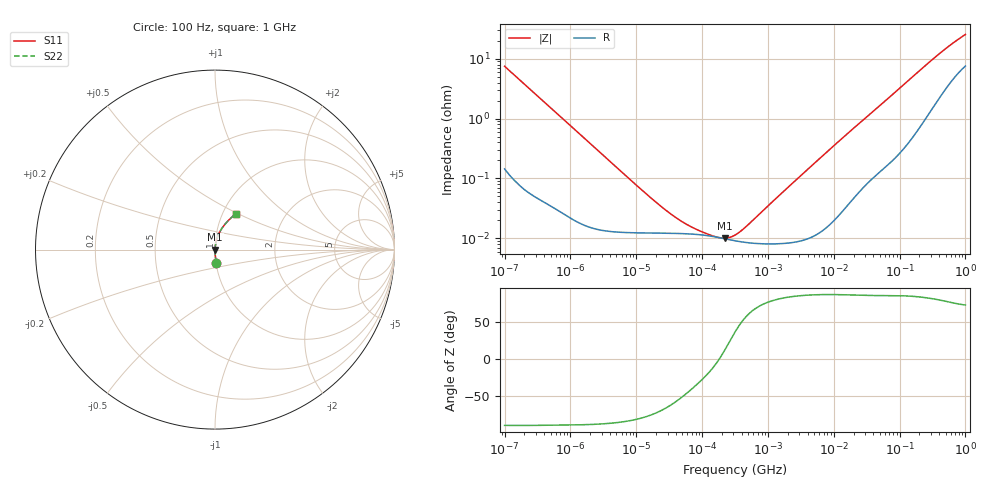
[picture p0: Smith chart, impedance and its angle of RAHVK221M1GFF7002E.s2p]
! RAHVK221M1GFF7002E  S-PARAMETER MODEL  (AEC-Q200 qualified)
! Model Generated by ELNA Corporation (http://www.ty-top.com)
! Version 1.0
! ELNA Control No. 201211
! Copyright (c) 2020 ELNA CO.,LTD. All Rights Reserved.
! Products Name : CONDUCTIVE POLYMER HYBRID ALUMINUM ELECTROLYTIC CAPACITORS
! Characteristics :
!  Capacitance  :  220uF  ,  Rated voltage  :  35V
!  Operating Temp. Range  :  -55 to +125 degC  ,  Endurance  :  4000hr at 125 degC
!  Dimension D  :  10mm  ,  Dimension L  :  8.7mm
! Frequency Range : 100Hz - 1GHz
! External Node Assignments :
!  1  o---| |---o  2
# MHz S RI R 50
!Freq[MHz].  S11 Real  S11 Imag  S21 Real  S21 Imag  S12 Real  S12 Imag  S22 Real  S22 Imag
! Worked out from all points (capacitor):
!   401 points, 100 Hz to 1 GHz, reference 50 ohm
!   read as one part in series: C = 213 uF near 108 Hz
!   lowest |Z| = 10.1 mohm at 220 kHz (marker M1)
!   series resonance near 181.9 kHz, so ESL is about 3.6 nH
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0.0001  0.00699 -0.0742  0.993 0.0742  0.993 0.0742  0.00699 -0.0742
0.000113  0.00558 -0.0659  0.9944 0.0659  0.9944 0.0659  0.00558 -0.0659
0.000309  0.00106 -0.0243  0.9989 0.0243  0.9989 0.0243  0.00106 -0.0243
0.001488  0.000198 -0.00513  0.9998 0.00513  0.9998 0.00513  0.000198 -0.00513
0.009495  0.000124 -0.000806  0.9999 0.000806  0.9999 0.000806  0.000124 -0.000806
0.022131  0.000122 -0.000343  0.9999 0.000343  0.9999 0.000343  0.000122 -0.000343
0.040504  0.000121 -0.000183  0.9999 0.000183  0.9999 0.000183  0.000121 -0.000183
0.071203  0.000118 -9.63e-05  0.9999 9.63e-05  0.9999 9.63e-05  0.000118 -9.63e-05
0.141254  0.000108 -2.52e-05  0.9999 2.52e-05  0.9999 2.52e-05  0.000108 -2.52e-05
0.179887  0.000103 -1.15e-06  0.9999 1.15e-06  0.9999 1.15e-06  0.000103 -1.15e-06
0.220039  9.85e-05 2.07e-05  0.9999 -2.07e-05  0.9999 -2.07e-05  9.85e-05 2.07e-05
0.269153  9.41e-05 4.51e-05  0.9999 -4.51e-05  0.9999 -4.51e-05  9.41e-05 4.51e-05
0.316228  9.1e-05 6.71e-05  0.9999 -6.71e-05  0.9999 -6.71e-05  9.1e-05 6.71e-05
0.371535  8.82e-05 9.18e-05  0.9999 -9.18e-05  0.9999 -9.18e-05  8.82e-05 9.18e-05
0.473151  8.49e-05 0.000135  0.9999 -0.000135  0.9999 -0.000135  8.49e-05 0.000135
4.704354  0.000108 0.00166  0.9999 -0.00166  0.9999 -0.00166  0.000108 0.00166
15.75796  0.000371 0.00546  0.9996 -0.00546  0.9996 -0.00546  0.000371 0.00546
69.9842  0.00228 0.0225  0.9977 -0.0225  0.9977 -0.0225  0.00228 0.0225
169.8244  0.00816 0.0527  0.9918 -0.0527  0.9918 -0.0527  0.00816 0.0527
380.1894  0.0317 0.1078  0.9683 -0.1078  0.9683 -0.1078  0.0317 0.1078
641.9482  0.0691 0.1565  0.9309 -0.1565  0.9309 -0.1565  0.0691 0.1565
1000  0.1152 0.1996  0.8848 -0.1996  0.8848 -0.1996  0.1152 0.1996
